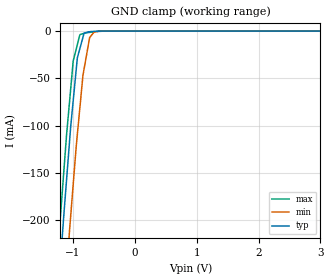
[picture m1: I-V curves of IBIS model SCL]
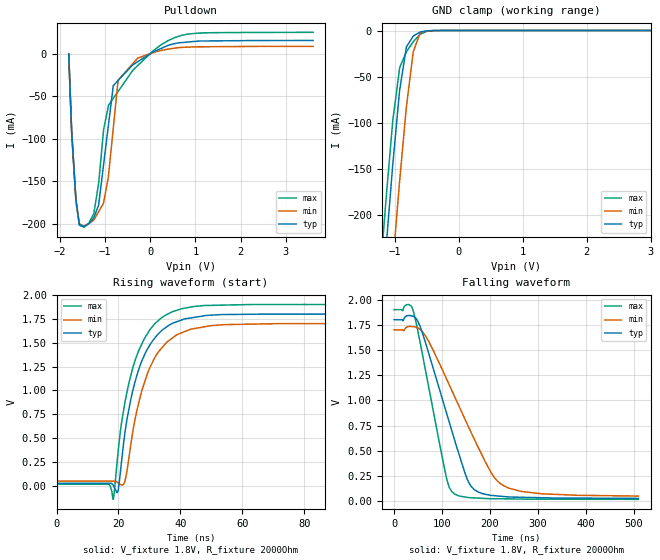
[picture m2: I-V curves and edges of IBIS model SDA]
|Texas Instruments Incorporated
|Ultra low power, High performance DirectPath Class-G headphone amplifier
| Marketing part#   Voltage Range(Digital)   Package-type   #pin
|TPA2028D1YFFR   1.7V to 1.9V   DSBGA   9
|TPA2028D1YFFT   1.7V to 1.9V   DSBGA   9
[IBIS Ver]   4.0
[File name]   tpa2028d1.ibs
[File Rev]   1.0
[Date]   03/20/2012
[Source]   Texas Instruments Incorporated.
   Analog-eLab, HPA
   12500 TI Blvd
   Dallas, TX -75243
   For Support e-mail: elab_ibis@list.ti.com
[Notes]   Revision History:
   1.0: 03/20/2012
   - Initial version of the model
   - Initial Model generated from simulations.
   - Model not matched to measurements
   - ccomp values are based on PVT conditions although listed
   in numerical order
   - Pull dowon non-monotinicity in SDA reflects
   the behavior based on simulations
[Disclaimer]
 This product is designed as an aid for customers of Texas Instruments.
 No warranties, either expressed or implied, with respect to this third
 party software (if any) or with respect to its fitness for any
 particular purpose is claimed by Texas Instruments or the author. The
 software (if any) is provided solely on an "as is" basis. The entire
 risk as to its quality and performance is with the customer
[Copyright] (C) Copyright 2012 Texas Instruments Incorporated.
   All rights reserved.
|   PCM5101
[Component]   tpa2028d1
[Manufacturer] TI
[Package]   | 20 pin  package
| variable   typ   min   max
R_pkg   0.01   0.008   0.012
L_pkg   0.1nH   0.08nH   0.12nH
C_pkg   0.1pF   0.08pF   0.12pF
|-------------------------PIN------------------------------------------------
[Pin] signal_name  model_name  R_pin  L_pin C_pin
A1   PGND   GND   NA   NA   NA
A2   SCL   SCL   NA   NA   NA
A3   SDA   SDA   NA   NA   NA
B1   OUT+   TERM   NA   NA   NA
B2   EN   SCL   NA   NA   NA
B3   IN+   TERM   NA   NA   NA
C1   OUT-   TERM   NA   NA   NA
C2   PVDD   POWER   NA   NA   NA
C3   IN-   TERM   NA   NA   NA
|   TERM Model
[Model] TERM
Model_type Terminator
C_comp   0   0   0
| variable   typ   min   max
[Voltage Range]   3.0V   2.5V   5.5V
[POWER Clamp Reference]  3.0V   2.5V   5.5V
[GND Clamp Reference]   0.0V   0.0V   5.5V
|Operating Temperature
[Temperature Range]   27   125   -25
| Models and submodels in the file (3): SCL (Input), SDA (I/O_open_drain), TERM (Terminator)
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|   SCL
[Model]   SCL
Model_type   Input
Vinl = 0.6
Vinh = 1.3
|   typ   min   max
C_comp   0.8513pF  0.8434pF   0.8631pF
[Voltage Range]   1.8   1.7   1.9
[Temperature Range]   27   125   -25
[Power Clamp Reference]   1.8   1.7   1.9
[GND Clamp Reference]   -0   -0   -0
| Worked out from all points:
|   GND clamp passes 1 mA (typ) near -0.76 V on its own axis
[GND Clamp]
|   Voltage   I(typ)   I(min)   I(max)
-1.8V     -811.2mA   -906.5mA   -765.4mA
-1.251V   -289.4mA   -387.3mA   -242.1mA
-1.21V    -252.1mA   -349.7mA   -204.1mA
-1.16V    -208mA     -305mA     -161.2mA
-1.052V   -116mA     -210mA     -74.15mA
-993.6mV  -73.3mA    -161.6mA   -31.3mA
-927mV    -28.2mA    -109.2mA   -14.29mA
-885.6mV  -18.3mA    -80.62mA   -3.713mA
-836.5mV  -6.553mA   -46.72mA   -2.709mA
-728.5mV  -681.4uA   -6.85mA    -1.349mA
-657.3mV  -289.1uA   -1.148mA   -754.1uA
3.6V      0A         0A         0A
[POWER Clamp]
|   Voltage   I(typ)   I(min)   I(max)
-1.8V     0A         0A         0A
0V        0A         0A         0A
3.6V      0A         0A         0A
|   SDA
[Model]   SDA
Model_type   I/O_open_drain
Polarity   Non-Inverting
Enable   Active-Low
Vinl = 0.6
Vinh = 1.3
Vmeas = 0.9
Vref = 1.8
Cref = 1pF
Rref = 2000
|   typ   min   max
C_comp   1.8117pF  1.637pF   1.945pF
[Voltage Range]   1.8   1.7   1.9
[Temperature Range]   27   125   -25
[Pullup Reference]   1.8   1.7   1.9
[Pulldown Reference]   -0   -0   -0
[Power Clamp Reference]   1.8   1.7   1.9
[GND Clamp Reference]   -0   -0   -0
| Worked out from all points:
|   slope of the pulldown table from 0 to 0.27 V, typ, clamps not added: 39.4 ohm
|   GND clamp passes 1 mA (typ) near -0.55 V on its own axis
|   falling waveform, V_fixture 1.8V, R_fixture 2000Ohm: 20-80 % time 67.4ns typ, 97.2ns min, 45.8ns max; typ from 1.8 V to 0.029 V
|   rising waveform, V_fixture 1.8V, R_fixture 2000Ohm: 20-80 % time 8.15ns typ, 8.47ns min, 8.09ns max; typ from 0.029 V to 1.8 V
[Pulldown]
|   Voltage   I(typ)   I(min)   I(max)
-1.8V     -657.3uA   -365.1uA   -967.5uA
-1.737V   -90.23mA   -89.87mA   -90.62mA
-1.641V   -171.8mA   -170.7mA   -173.4mA
-1.461V   -203.1mA   -202.3mA   -203.7mA
-1.245V   -192.6mA   -195.2mA   -187.6mA
-1.14V    -177.8mA   -185.5mA   -152.3mA
-1.029V   -129.9mA   -174.6mA   -89mA
-815.8mV  -37.59mA   -87.5mA    -52.53mA
-709mV    -31.55mA   -31.13mA   -44.38mA
-277mV    -9.53mA    -5.385mA   -14.11mA
788.8mV   13.35mA    7.467mA    22.46mA
3.6V      15.42mA    8.508mA    24.95mA
[GND Clamp]
|   Voltage   I(typ)   I(min)   I(max)
-1.8V     -863mA     -973.4mA   -809.4mA
-1.245V   -336.2mA   -448.4mA   -281.8mA
-1.141V   -241.9mA   -353.4mA   -188.9mA
-1.137V   -238.5mA   -349.9mA   -185.4mA
-1.029V   -145.6mA   -254mA     -97.84mA
-921.1mV  -64.7mA    -162.7mA   -40.19mA
-815.8mV  -17.72mA   -82.49mA   -23.13mA
-709mV    -6.043mA   -22.96mA   -12.14mA
-599.8mV  -1.571mA   -2.62mA    -4.124mA
-489.1mV  -253.7uA   -337.9uA   -588.8uA
-381.1mV  -26.99uA   -53.54uA   -40uA
3.6V      0A         0A         0A
[POWER Clamp]
|   Voltage   I(typ)   I(min)   I(max)
-1.8V     0A         0A         0A
0V        0A         0A         0A
3.6V      0A         0A         0A
[Ramp]
R_load = 2000
|   typ   min   max
dV/dt_r   1.06264/8.15583e-009  0.988797/8.46655e-009   1.12836/8.06205e-009
dV/dt_f   1.06269/6.71705e-008  0.988996/9.71727e-008   1.12837/4.57774e-008
[Falling Waveform]
V_fixture = 1.8V
V_fixture_min = 1.7V
V_fixture_max = 1.9V
R_fixture = 2000Ohm
C_fixture = 0F
|   Time   V(typ)   V(min)   V(max)
0s        1.8V       1.7V       1.9V
30.05ns   1.842V     1.732V     1.951V
40.36ns   1.834V     1.731V     1.884V
65.55ns   1.573V     1.64V      1.3V
108.7ns   888.8mV    1.222V     248.8mV
126.6ns   602.7mV    1.035V     71.17mV
161.1ns   146.2mV    680.3mV    35.35mV
200.1ns   59.9mV     304.4mV    26.17mV
229.2ns   46.98mV    152.9mV    24.42mV
510ns     28.84mV    51.63mV    19.38mV
[Rising Waveform]
V_fixture = 1.8V
V_fixture_min = 1.7V
V_fixture_max = 1.9V
R_fixture = 2000Ohm
C_fixture = 0F
|   Time   V(typ)   V(min)   V(max)
0s        28.92mV    51.96mV    19.39mV
16.94ns   28.69mV    51.58mV    18.97mV
18.27ns   10.37mV    51.55mV    -139.6mV
19.82ns   -55.35mV   34.66mV    333.9mV
22.05ns   545.7mV    45.39mV    862.8mV
26.44ns   1.208V     853.7mV    1.409V
29.3ns    1.429V     1.171V     1.591V
32.96ns   1.595V     1.406V     1.734V
44.03ns   1.763V     1.646V     1.878V
510ns     1.8V       1.7V       1.9V
